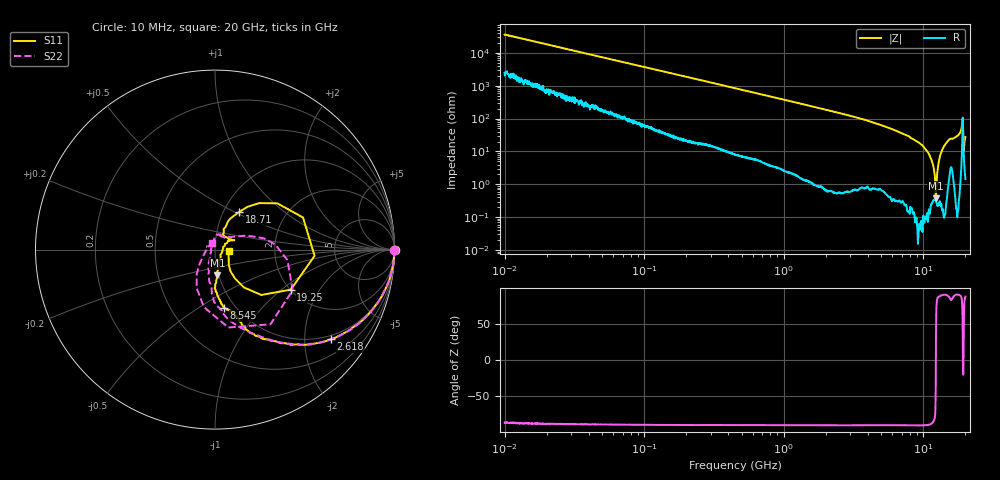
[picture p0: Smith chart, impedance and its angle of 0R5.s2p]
!Keysight Technologies,P5008B,MY61100088,A.16.20.02
!Date: Friday, August 30, 2024 10:34:22
!Correction: S11(C  2-Port  )
!S21(C  2-Port  )
!S12(C  2-Port  )
!S22(C  2-Port  )
!S2P File: Measurements: S11, S21, S12, S22:Log Frequency Sweep
# Hz S  dB  R 50
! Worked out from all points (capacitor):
!   1601 points, 10 MHz to 20 GHz, reference 50 ohm
!   read as one part in series: C = 444 fF near 10.39 MHz
!   lowest |Z| = 374 mohm at 12.32 GHz (marker M1)
!   series resonance near 12.29 GHz, so ESL is about 380 pH
!   S11 on the Smith chart (normalised r, x): 10 MHz: open; 2.618 GHz: 0.89, -2.66; 8.545 GHz: 0.89, -0.65; 18.71 GHz: 1.18, +0.53; 19.25 GHz: 2.01, -1.16; 20 GHz: 1.17, -0.02
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1e7  0.00 -0.2  -51.04 85.9  -51.08 86.4  -0.00 -0.2
3.555162e7  -0.00 -0.6  -40.17 87.8  -40.19 87.7  -0.00 -0.6
1.263918e8  -0.01 -2.1  -29.35 87.1  -29.35 87.1  -0.01 -2.1
4.472136e8  -0.08 -7.2  -18.52 82.2  -18.53 82.2  -0.07 -7.3
9.473091e8  -0.28 -14.9  -12.25 74.6  -12.26 74.6  -0.29 -15.1
1.589917e9  -0.73 -24.2  -8.18 65.4  -8.19 65.4  -0.74 -24.5
2.61821e9  -1.76 -37.7  -4.82 52.0  -4.82 52.0  -1.76 -37.8
3.995989e9  -3.50 -52.0  -2.63 37.6  -2.64 37.5  -3.50 -51.7
5.652411e9  -5.91 -66.8  -1.31 22.8  -1.31 22.8  -5.93 -66.6
8.545299e9  -9.66 -81.1  -0.48 6.1  -0.48 6.0  -9.67 -85.3
1.093983e10  -12.96 -89.2  -0.20 -3.4  -0.21 -3.5  -12.90 -94.7
1.231939e10  -16.84 -84.7  -0.07 -8.3  -0.07 -8.4  -16.97 -105.2
1.291876e10  -20.42 -77.7  0.00 -10.7  -0.00 -10.9  -21.01 -113.5
1.361179e10  -27.49 -45.2  0.05 -13.8  0.05 -13.9  -30.49 -141.8
1.400536e10  -27.70 -2.8  0.07 -15.6  0.07 -15.8  -33.34 145.3
1.540129e10  -19.51 33.1  -0.14 -22.2  -0.14 -22.4  -21.22 76.7
1.75924e10  -20.67 59.5  -0.01 -30.4  -0.01 -30.6  -21.44 54.2
1.827386e10  -17.24 65.2  -0.12 -36.0  -0.12 -36.2  -17.60 33.6
1.871311e10  -12.06 57.3  -0.57 -43.3  -0.57 -43.5  -12.46 17.4
1.898171e10  -7.27 36.5  -2.38 -52.5  -2.39 -52.7  -7.80 -8.2
1.925417e10  -6.42 -27.8  -4.28 -12.5  -4.28 -12.7  -7.13 -80.4
2e10  -22.29 -5.8  -0.13 -31.0  -0.13 -31.2  -27.32 116.5
